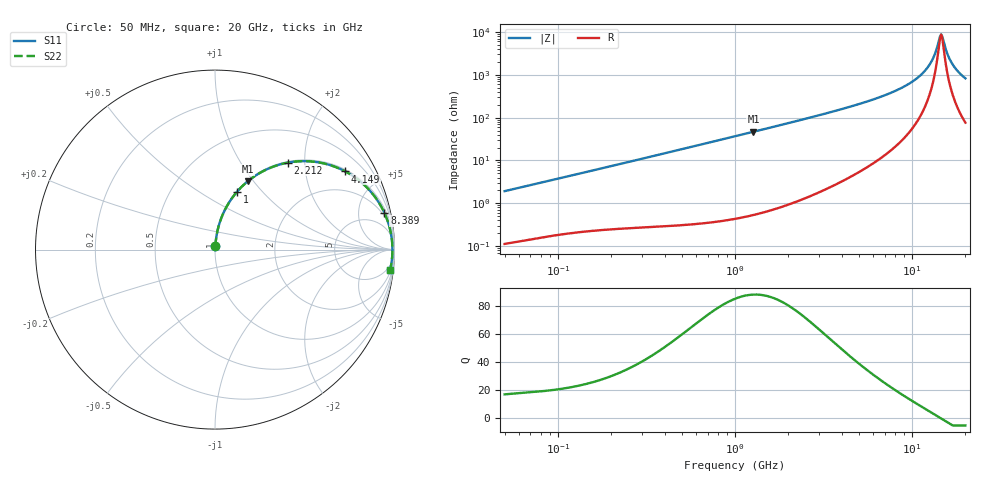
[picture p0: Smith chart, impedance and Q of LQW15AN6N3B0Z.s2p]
!Murata Part Number: LQW15AN6N3B0Z
!These Parameters are Measured in Series Mode Connection
!  o--[Z]--o
!Port1  Port2
!  o-------o
!Freq. Start=50[MHz] Stop=20[GHz], 401[Steps]
# Hz S RI R 50
!Freq.(Hz) S11(Real) S11(Imag) S21(Real) S21(Imag) S12(Real) S12(Imag) S22(Real) S22(Imag)
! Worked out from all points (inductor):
!   401 points, 50 MHz to 20 GHz, reference 50 ohm
!   read as one part in series: L = 6.06 nH near 51.52 MHz
!   highest Q = 87.7 at 1.271 GHz (marker M1), where L = 5.85 nH
!   self-resonance near 14.39 GHz
!   S11 on the Smith chart (normalised r, x): 50 MHz: 1.00, +0.04; 1 GHz: 1.01, +0.73; 2.212 GHz: 1.02, +1.65; 4.149 GHz: 1.07, +3.29; 8.389 GHz: 1.49, +9.12; 20 GHz: 3, -16
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5e7  0.00149 0.0191  0.9985 -0.0191  0.9985 -0.0191  0.00149 0.0191
1.364002e8  0.00469 0.0504  0.9953 -0.0504  0.9953 -0.0504  0.00469 0.0504
3.721004e8  0.021 0.1331  0.979 -0.1331  0.979 -0.1331  0.021 0.1331
1e9  0.1215 0.3209  0.8785 -0.3209  0.8785 -0.3209  0.1215 0.3209
1.270815e9  0.1821 0.3803  0.8179 -0.3803  0.8179 -0.3803  0.1821 0.3803
2.211938e9  0.4069 0.4848  0.5931 -0.4848  0.5931 -0.4848  0.4069 0.4848
2.728004e9  0.5154 0.4924  0.4846 -0.4924  0.4846 -0.4924  0.5154 0.4924
4.149438e9  0.7265 0.4353  0.2735 -0.4353  0.2735 -0.4353  0.7265 0.4353
5.683258e9  0.8493 0.3431  0.1507 -0.3431  0.1507 -0.3431  0.8493 0.3431
7.442007e9  0.9214 0.2481  0.0786 -0.2481  0.0786 -0.2481  0.9214 0.2481
8.389408e9  0.9442 0.2041  0.0558 -0.2041  0.0558 -0.2041  0.9442 0.2041
1.034674e10  0.972 0.1265  0.028 -0.1265  0.028 -0.1265  0.972 0.1265
1.201863e10  0.9834 0.0713  0.0166 -0.0713  0.0166 -0.0713  0.9834 0.0713
1.314879e10  0.9871 0.0383  0.0129 -0.0383  0.0129 -0.0383  0.9871 0.0383
1.354865e10  0.9879 0.0273  0.0121 -0.0273  0.0121 -0.0273  0.9879 0.0273
1.417136e10  0.9885 0.0108  0.0115 -0.0108  0.0115 -0.0108  0.9885 0.0108
1.460232e10  0.9887 -0.000229  0.0113 0.000229  0.0113 0.000229  0.9887 -0.000229
1.504638e10  0.9886 -0.0112  0.0114 0.0112  0.0114 0.0112  0.9886 -0.0112
1.597544e10  0.9876 -0.0332  0.0124 0.0332  0.0124 0.0332  0.9876 -0.0332
1.696185e10  0.9857 -0.0553  0.0143 0.0553  0.0143 0.0553  0.9857 -0.0553
1.828096e10  0.9819 -0.0829  0.0181 0.0829  0.0181 0.0829  0.9819 -0.0829
2e10  0.9751 -0.1161  0.0249 0.1161  0.0249 0.1161  0.9751 -0.1161
